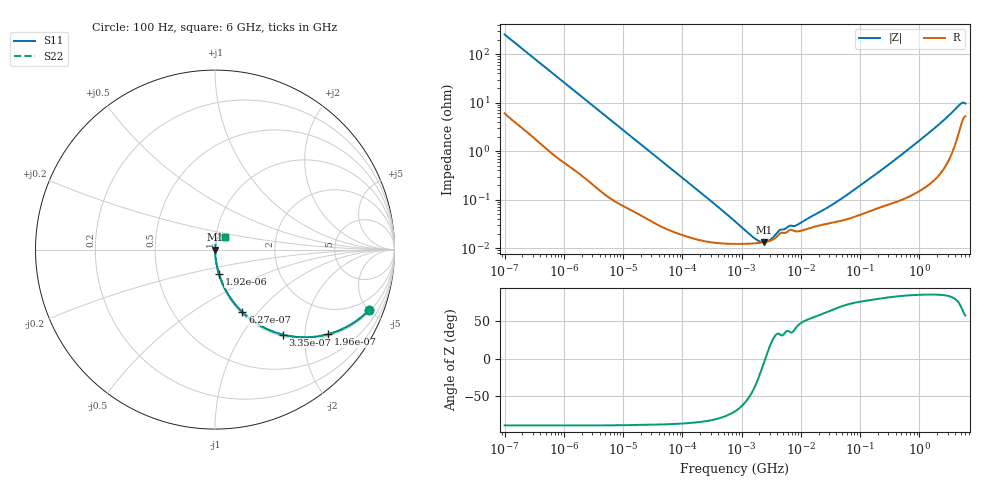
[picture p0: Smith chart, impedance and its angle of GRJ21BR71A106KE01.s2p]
!Murata Part Number: GRJ21BR71A106KE01
!These Parameters are Measured in Series Mode Connection
!Data Generated on Jun 19, 2026
!  o--ll--o
!Port1  Port2
!  o------o
!Operation Temp=25[degC], DC Bias Voltage=0[V]
!Freq. Start=100[Hz] Stop=6[GHz] 401[Steps]
# Hz S RI R 50
!Freq.(Hz) S11(Real) S11(Imag) S21(Real) S21(Imag) S12(Real) S12(Imag) S22(Real) S22(Imag)
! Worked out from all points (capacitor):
!   401 points, 100 Hz to 6 GHz, reference 50 ohm
!   read as one part in series: C = 6.23 uF near 109 Hz
!   lowest |Z| = 13.3 mohm at 2.373 MHz (marker M1)
!   series resonance near 2.51 MHz, so ESL is about 650 pH
!   S11 on the Smith chart (normalised r, x): 100 Hz: 1.12, -5.09; 196 Hz: 1.06, -2.62; 335 Hz: 1.03, -1.55; 627 Hz: 1.02, -0.83; 1.92 kHz: 1.01, -0.28; 6 GHz: 1.10, +0.16
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100  0.8605 -0.3349  0.1395 0.3349  0.1395 0.3349  0.8605 -0.3349
196  0.6297 -0.4715  0.3703 0.4715  0.3703 0.4715  0.6297 -0.4715
335  0.3767 -0.4734  0.6233 0.4734  0.6233 0.4734  0.3767 -0.4734
627  0.153 -0.3494  0.847 0.3494  0.847 0.3494  0.153 -0.3494
1026  0.0661 -0.2376  0.9339 0.2376  0.9339 0.2376  0.0661 -0.2376
1920  0.0218 -0.1346  0.9782 0.1346  0.9782 0.1346  0.0218 -0.1346
2008  0.0201 -0.129  0.9799 0.129  0.9799 0.129  0.0201 -0.129
6433  0.00276 -0.0417  0.9972 0.0417  0.9972 0.0417  0.00276 -0.0417
40335  0.000341 -0.00687  0.9997 0.00687  0.9997 0.00687  0.000341 -0.00687
774597  0.000123 -0.000336  0.9999 0.000336  0.9999 0.000336  0.000123 -0.000336
1658239  0.000126 -9.84e-05  0.9999 9.84e-05  0.9999 9.84e-05  0.000126 -9.84e-05
2372521  0.000132 -1.31e-05  0.9999 1.31e-05  0.9999 1.31e-05  0.000132 -1.31e-05
3103719  0.000144 5.07e-05  0.9999 -5.07e-05  0.9999 -5.07e-05  0.000144 5.07e-05
4440638  0.000201 0.000126  0.9998 -0.000126  0.9998 -0.000126  0.000201 0.000126
6353432  0.000233 0.00017  0.9998 -0.00017  0.9998 -0.00017  0.000233 0.00017
8311524  0.000222 0.000194  0.9998 -0.000194  0.9998 -0.000194  0.000222 0.000194
1.555665e7  0.000269 0.000373  0.9997 -0.000373  0.9997 -0.000373  0.000269 0.000373
4.764863e7  0.000368 0.000965  0.9996 -0.000965  0.9996 -0.000965  0.000368 0.000965
3.124326e8  0.000829 0.00536  0.9992 -0.00536  0.9992 -0.00536  0.000829 0.00536
1.712697e9  0.00318 0.0279  0.9968 -0.0279  0.9968 -0.0279  0.00318 0.0279
4.796499e9  0.0336 0.0814  0.9664 -0.0814  0.9664 -0.0814  0.0336 0.0814
6e9  0.0552 0.0729  0.9448 -0.0729  0.9448 -0.0729  0.0552 0.0729
